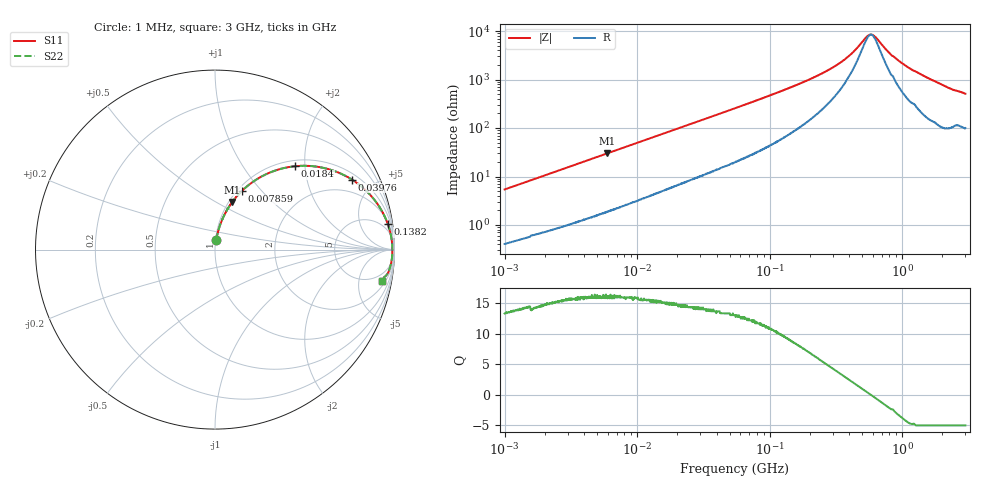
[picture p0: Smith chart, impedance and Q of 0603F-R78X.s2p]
!s-Parameter Generated by FASTRON Sdn. Bhd.
!FASTRON P/N : 0603F-R78X
!Keysight Technologies: E4991B_MY54100416_A.01.15
!Date: Thu Jun 20 13:33:53 2024
!Version  :Rev00  Thu Jun 20 13:33:53 2024
!Data & Calibration Information:
!Freq  S11  S21  S12  S22
!PortZ  Port1:50+j0  Port2:50+j0
!When reading reference impedance value at option line is always used.
! Remarks : This data is being provided solely for informational purposes.
# Hz S dB R 50
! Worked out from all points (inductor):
!   1601 points, 1 MHz to 3 GHz, reference 50 ohm
!   read as one part in series: L = 848 nH near 1.041 MHz
!   highest Q = 16.1 at 5.938 MHz (marker M1), where L = 802 nH
!   self-resonance near 580.9 MHz
!   S11 on the Smith chart (normalised r, x): 1 MHz: 1.01, +0.11; 7.859 MHz: 1.05, +0.78; 18.4 MHz: 1.12, +1.78; 39.76 MHz: 1.28, +3.74; 138.2 MHz: 2, +13; 3 GHz: 3, -10
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1000000  -25.40 82.6  -0.05 -3.1  -0.05 -3.1  -25.40 82.6
3804036  -14.50 75.5  -0.26 -10.9  -0.26 -10.9  -14.50 75.5
5938264  -11.00 70.1  -0.52 -16.4  -0.52 -16.4  -11.00 70.1
7858845  -8.93 65.5  -0.80 -20.9  -0.80 -20.9  -8.93 65.5
1.447069e7  -5.04 52.3  -2.02 -34.0  -2.02 -34.0  -5.04 52.3
1.839937e7  -3.82 46.2  -2.82 -40.0  -2.82 -40.0  -3.82 46.2
2.637991e7  -2.41 36.9  -4.41 -49.1  -4.41 -49.1  -2.41 36.9
3.976269e7  -1.35 27.1  -6.79 -58.7  -6.79 -58.7  -1.35 27.1
5.504702e7  -0.83 20.6  -9.04 -65.0  -9.04 -65.0  -0.83 20.6
1.382301e8  -0.24 8.4  -16.60 -75.3  -16.60 -75.3  -0.24 8.4
2.083556e8  -0.16 5.2  -20.70 -76.1  -20.70 -76.1  -0.16 5.2
2.898922e8  -0.13 3.3  -24.60 -74.1  -24.60 -74.1  -0.13 3.3
3.631036e8  -0.11 2.1  -28.10 -69.7  -28.10 -69.7  -0.11 2.1
4.304467e8  -0.11 1.3  -31.60 -61.4  -31.60 -61.4  -0.11 1.3
5.337858e8  -0.10 0.4  -37.50 -28.6  -37.50 -28.6  -0.10 0.4
5.696638e8  -0.10 0.1  -38.60 -7.2  -38.60 -7.2  -0.10 0.1
6.264832e8  -0.10 -0.3  -37.70 26.5  -37.70 26.5  -0.10 -0.3
7.925923e8  -0.10 -1.4  -31.30 63.2  -31.30 63.2  -0.10 -1.4
9.828732e8  -0.11 -2.4  -27.10 72.2  -27.10 72.2  -0.11 -2.4
1.194682e9  -0.13 -3.5  -24.10 74.6  -24.10 74.6  -0.13 -3.5
2.188818e9  -0.26 -8.0  -17.10 73.9  -17.10 73.9  -0.26 -8.0
3e9  -0.47 -10.5  -14.60 68.2  -14.60 68.2  -0.47 -10.5
